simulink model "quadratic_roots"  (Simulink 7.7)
settings: Solver=VariableStepDiscrete  StartTime=0.0  StopTime=10.0  RelTol=1e-3

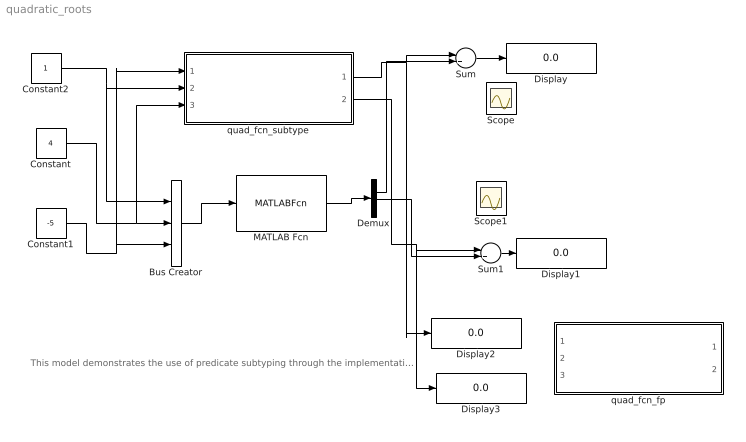
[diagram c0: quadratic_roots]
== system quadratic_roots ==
  note: This model demonstrates the use of predicate subtyping through the implementation of quad_fcn, which will give the real roots of a quadratic function. results are compared to the matlab function roots, results are generally the same, although sometimes there is a small error on the order of 1e-16. Currently does not activly check that inputs satisfy subtype constraints, in these cases proper output is not guaranteed. This example will not work under CVC3 as complex functions like sqrt are not supported. This example requires the NASA PVS libraries
  Bus Creator : BusCreator  Inputs=3
  Constant : Constant  Value=4
  Constant1 : Constant  Value=-5
  Constant2 : Constant
  Demux : Demux  Outputs=2
  Display{,1..3} (4 alike) : Display
  MATLAB Fcn : MATLABFcn  MATLABFcn=roots  OutputDimensions=2  Output1D=off
  Scope : Scope
  Scope1 : Scope
  Sum : Sum  Inputs=|+-
  Sum1 : Sum  Inputs=|+-
  quad_fcn_fp : Subsystem
  quad_fcn_subtype : Subsystem
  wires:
  Constant2/1 -> Bus Creator/1, quad_fcn_subtype/2(a)
  Constant/1 -> Bus Creator/2, quad_fcn_subtype/3(b)
  Constant1/1 -> Bus Creator/3, quad_fcn_subtype/1(c)
  Bus Creator/1 -> MATLAB Fcn/1
  MATLAB Fcn/1 -> Demux/1
  quad_fcn_subtype/1(x1) -> Sum/1, Display2/1
  Demux/2 -> Sum1/2
  quad_fcn_subtype/2(x2) -> Sum1/1, Display3/1
  Sum1/1 -> Display1/1
  Sum/1 -> Display/1
  Demux/1 -> Sum/2

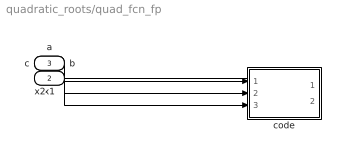
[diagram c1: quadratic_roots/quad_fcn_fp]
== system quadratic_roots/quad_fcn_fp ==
  a : Inport
  b : Inport  Port=2
  c : Inport  Port=3
  code : Stateflow chart  TreatAsAtomicUnit=on
  x1 : Outport
  x2 : Outport  Port=2
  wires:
  a/1 -> code/1(a)
  b/1 -> code/2(b)
  c/1 -> code/3(c)
  code/1(x1) -> x1/1
  code/2(x2) -> x2/1

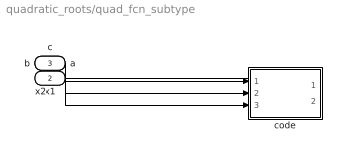
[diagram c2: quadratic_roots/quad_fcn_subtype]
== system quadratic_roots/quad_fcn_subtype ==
  c : Inport
  a : Inport  Port=2
  b : Inport  Port=3
  code : Stateflow chart  TreatAsAtomicUnit=on
  x1 : Outport
  x2 : Outport  Port=2
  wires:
  c/1 -> code/1(c)
  a/1 -> code/2(a)
  b/1 -> code/3(b)
  code/1(x1) -> x1/1
  code/2(x2) -> x2/1

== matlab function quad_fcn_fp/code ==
function [x1,x2] = quad_fcn_fp(a,b,c)
%%#eml
x1=-c/b;
x2=NaN;
if(a == 0)
  if(b ~= 0)
    x1 = -c/b;
    x2 = NaN;
  elseif(b == 0)
    x1 = NaN;
    x2 = NaN;
  end
elseif(a ~= 0)
  if((b*b) - 4*a*c == 0)
    x1 = -b/2*a;
    x2 = NaN;
  elseif((b*b) - 4*a*c < 0)
    x1 = NaN;
    x2 = NaN;
  elseif((b*b) - 4*a*c > 0)
    if(b >= 0)
      x1 = (-b - sqrt(b*b - 4*a*c)) / 2*a;
      x2 = c / (a* ((-b - sqrt(b*b - 4*a*c)) / 2*a));
    elseif(b < 0)
      x1 = (-b + sqrt(b*b - 4*a*c)) / 2*a;
      x2 = c / (a* ((-b + sqrt(b*b - 4*a*c)) / 2*a));
    end
  end
end

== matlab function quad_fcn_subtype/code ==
function [x1,x2] = quad_fcn_subtype(c,a,b)
%%#eml
x1=-c/b;
x2=-c/b;
if(a == 0)
  if(b ~= 0)
    x1 = -c/b;
    x2 = -c/b;
  end
elseif(a ~= 0)
  if((b^2) - 4*a*c == 0)
    x1 = -b/2*a;
    x2 = -b/2*a;
  elseif((b^2) - 4*a*c > 0)
    if(b>=0)
      x1 = (-b - sqrt(b^2 - 4*a*c)) / 2*a;
      x2 = c / (a* ((-b - sqrt(b^2 - 4*a*c)) / 2*a));
    elseif(b<0)
      x1 = (-b + sqrt(b^2 - 4*a*c)) / 2*a;
      x2 = c / (a* ((-b + sqrt(b^2 - 4*a*c)) / 2*a));
    end
  end
end
